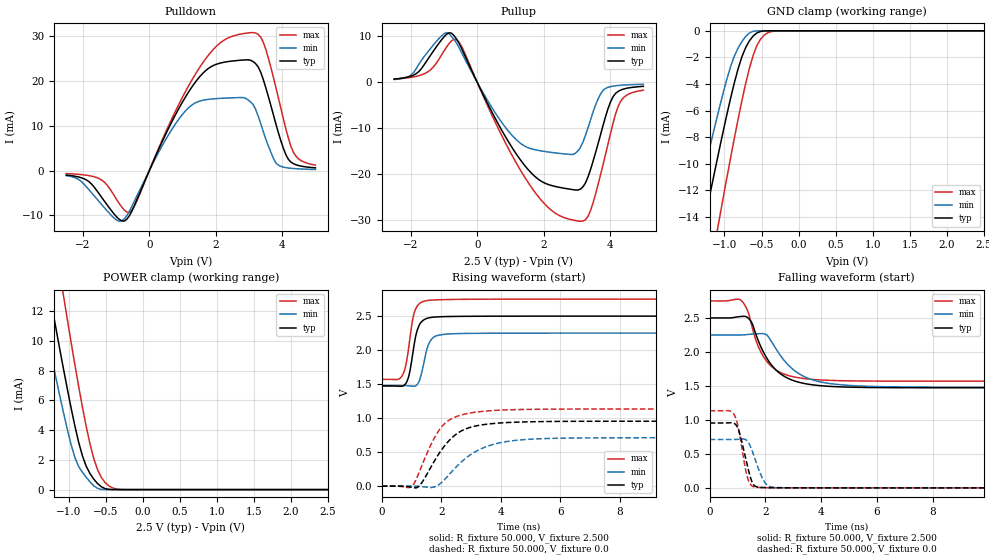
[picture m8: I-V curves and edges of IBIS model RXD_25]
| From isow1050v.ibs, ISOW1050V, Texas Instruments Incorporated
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|   RXD_25 Model
[Model] RXD_25
Model_type 3-state
Polarity   Non-Inverting
Enable   Active-High
C_comp   2.100pF   1.700pF   2.500pF
[Temperature Range]   27.000   -40.000   0.125k
[Voltage Range]   2.500V   2.250V   2.750V
[Pullup Reference]   2.500V   2.250V   2.750V
[Pulldown Reference]   0.0V   0.0V   0.0V
[POWER Clamp Reference]   2.500V   2.250V   2.750V
[GND Clamp Reference]   0.0V   0.0V   0.0V
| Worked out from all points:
|   slope of the pulldown table from 0 to 0.375 V, typ, clamps not added: 59.9 ohm
|   slope of the pullup table from 0 to 0.375 V, typ, clamps not added: 67.9 ohm
|   GND clamp passes 1 mA (typ) near -0.69 V on its own axis
|   POWER clamp passes 1 mA (typ) near -0.70 V on its own axis
|   rising waveform, R_fixture 50.000, V_fixture 2.500: 20-80 % time 256ps typ, 262ps min, 248ps max; typ from 1.47 V to 2.5 V
|   rising waveform, R_fixture 50.000, V_fixture 0.0: 20-80 % time 962ps typ, 1.24ns min, 806ps max; typ from 0 V to 0.954 V
|   falling waveform, R_fixture 50.000, V_fixture 2.500: 20-80 % time 912ps typ, 1.11ns min, 737ps max; typ from 2.5 V to 1.47 V
|   falling waveform, R_fixture 50.000, V_fixture 0.0: 20-80 % time 335ps typ, 392ps min, 295ps max; typ from 0.954 V to 0 V
[Pulldown]
|Voltage   I(typ)   I(min)   I(max)
-2.5V     -1.006mA   -1.146mA   -683.4uA
-1.816V   -2.489mA   -4.292mA   -1.135mA
-980mV    -10.37mA   -11.08mA   -6.513mA
-600mV    -10.08mA   -9.1mA     -9.329mA
1.224V    18.01mA    14.29mA    19.46mA
2.136V    23.98mA    16.1mA     28.49mA
3.048V    24.6mA     15.29mA    30.77mA
3.428V    20.34mA    8.751mA    28.66mA
3.808V    10.42mA    1.717mA    18.56mA
4.188V    2.466mA    561.4uA    7.144mA
4.492V    1.114mA    374uA      2.605mA
5V        603.7uA    241uA      1.209mA
[Pullup]
|Voltage   I(typ)   I(min)   I(max)
-2.5V     726.9uA    631.1uA    715.4uA
-1.764V   2.329mA    3.88mA     1.453mA
-1.004V   9.893mA    10.58mA    6.798mA
-624mV    9.443mA    8.566mA    9.327mA
1.276V    -16.63mA   -13.11mA   -18.81mA
2.188V    -22.34mA   -15.2mA    -27.56mA
3.1V      -23.25mA   -14.19mA   -30.23mA
3.404V    -19.09mA   -8.301mA   -28.02mA
3.708V    -11.45mA   -2.567mA   -20.2mA
4.088V    -3.112mA   -806uA     -8.857mA
4.392V    -1.468mA   -581.7uA   -3.395mA
5V        -853.6uA   -412.7uA   -1.687mA
[GND_clamp]
|Voltage   I(typ)   I(min)   I(max)
-2.5V     -49.36mA   -40.8mA    -60.78mA
-1.48V    -20.2mA    -15.54mA   -27.23mA
-1.429V   -18.76mA   -14.3mA    -25.58mA
-1.276V   -14.51mA   -10.62mA   -20.67mA
-1.072V   -8.986mA   -5.867mA   -14.25mA
-868mV    -3.938mA   -1.917mA   -8.115mA
-766mV    -1.977mA   -816.7uA   -5.29mA
-664mV    -757.7uA   -164uA     -2.832mA
-562mV    -158.3uA   -4.791uA   -1.109mA
-511mV    -45.93uA   -437.2nA   -609.9uA
-358mV    -238.8nA   -170.8pA   -47.56uA
2.5V      0A         0A         -857.3pA
[POWER_clamp]
|Voltage   I(typ)   I(min)   I(max)
-2.5V     48.98mA    40.5mA     60.37mA
-1.427V   17.97mA    13.67mA    24.5mA
-1.376V   16.53mA    12.42mA    22.84mA
-1.274V   13.68mA    9.95mA     19.53mA
-1.223V   12.27mA    8.731mA    17.9mA
-1.07V    8.13mA     5.188mA    13.07mA
-917mV    4.315mA    2.178mA    8.444mA
-815mV    2.287mA    1.173mA    5.584mA
-611mV    414.1uA    85.69uA    1.354mA
-458mV    17.92uA    162.2nA    253.4uA
-305mV    107.2nA    59.5pA     15.5uA
2.5V      0A         0A         0A
[Ramp]
| variable   typ   min   max
dV/dt_r   0.573/0.962n   0.427/1.238n   0.681/0.806n
dV/dt_f   0.617/0.911n   0.462/1.104n   0.708/0.736n
R_load = 50.000
[Rising Waveform]
R_fixture= 50.000
V_fixture= 2.500
V_fixture_min= 2.250
V_fixture_max= 2.750
|time   V(typ)   V(min)   V(max)
0s        1.472V     1.48V      1.569V
605ps     1.469V     1.48V      1.582V
813ps     1.513V     1.477V     1.787V
944ps     1.687V     1.473V     2.168V
1.093ns   2.092V     1.469V     2.552V
1.265ns   2.372V     1.552V     2.683V
1.484ns   2.461V     1.955V     2.726V
1.734ns   2.485V     2.185V     2.737V
2.344ns   2.495V     2.24V      2.745V
15ns      2.5V       2.25V      2.75V
[Rising Waveform]
R_fixture= 50.000
V_fixture= 0.0
V_fixture_min= 0.0
V_fixture_max= 0.0
|time   V(typ)   V(min)   V(max)
0s        289.5nV    183.8nV    809.3nV
1.02ns    -18.15mV   280.3uV    -1.282mV
1.318ns   33.6mV     -6.419mV   268.9mV
1.697ns   314mV      -19.23mV   648.7mV
1.997ns   525mV      47.41mV    864.1mV
2.482ns   757mV      273.2mV    1.018V
2.994ns   866.3mV    465mV      1.076V
3.844ns   924.1mV    624.5mV    1.114V
5.184ns   947.6mV    693.9mV    1.13V
15ns      954.4mV    711.6mV    1.134V
[Falling Waveform]
R_fixture= 50.000
V_fixture= 2.500
V_fixture_min= 2.250
V_fixture_max= 2.750
|time   V(typ)   V(min)   V(max)
0s        2.5V       2.25V      2.75V
1.145ns   2.522V     2.25V      2.751V
1.493ns   2.442V     2.261V     2.415V
1.731ns   2.18V      2.267V     2.095V
2.011ns   1.935V     2.259V     1.882V
2.476ns   1.698V     1.984V     1.711V
3.106ns   1.565V     1.707V     1.626V
3.926ns   1.505V     1.563V     1.589V
5.236ns   1.48V      1.501V     1.573V
15ns      1.472V     1.48V      1.569V
[Falling Waveform]
R_fixture= 50.000
V_fixture= 0.0
V_fixture_min= 0.0
V_fixture_max= 0.0
|time   V(typ)   V(min)   V(max)
0s        954.4mV    711.6mV    1.134V
678ps     956.3mV    711.2mV    1.136V
881ps     947.5mV    711.8mV    1.075V
1.057ns   828.2mV    714.9mV    823mV
1.351ns   331.4mV    688.7mV    161mV
1.502ns   105.7mV    568.5mV    34.34mV
1.612ns   31.3mV     442.4mV    12.7mV
1.958ns   3.81mV     93.27mV    3.288mV
2.308ns   1.5mV      7.276mV    1.469mV
15ns      567pV      821.9pV    102.9nV
